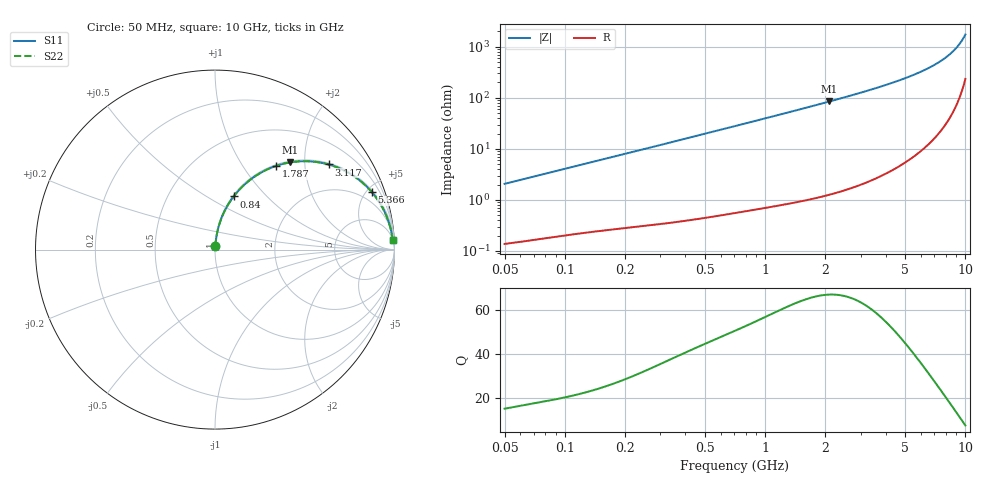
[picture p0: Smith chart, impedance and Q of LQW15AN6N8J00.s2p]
!Murata Part Number: LQW15AN6N8J00
!These Parameters are Measured in Series Mode Connection
!  o--[Z]--o
!Port1  Port2
!  o-------o
!Freq. Start=50[MHz] Stop=10[GHz], 401[Steps]
# Hz S RI R 50
!Freq.(Hz)	S 11(Real)	S 11(Imag)	S 21(Real)	S 21(Imag)	S 12(Real)	S 12(Imag)	S 22(Real)	S 22(Imag)
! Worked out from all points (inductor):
!   401 points, 50 MHz to 10 GHz, reference 50 ohm
!   read as one part in series: L = 6.54 nH near 51.34 MHz
!   highest Q = 67 at 2.095 GHz (marker M1), where L = 6.45 nH
!   S11 on the Smith chart (normalised r, x): 50 MHz: 1.00, +0.04; 840 MHz: 1.01, +0.66; 1.787 GHz: 1.02, +1.44; 3.117 GHz: 1.04, +2.64; 5.366 GHz: 1.13, +5.40; 10 GHz: 6, +35
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5e7  0.0018 0.0206  0.9982 -0.0206  0.9982 -0.0206  0.0018 0.0206
1.214486e8  0.00462 0.0487  0.9954 -0.0487  0.9954 -0.0487  0.00462 0.0487
2.949953e8  0.0168 0.115  0.9832 -0.115  0.9832 -0.115  0.0168 0.115
4.628099e8  0.0364 0.1761  0.9636 -0.1761  0.9636 -0.1761  0.0364 0.1761
7.071068e8  0.077 0.2568  0.923 -0.2568  0.923 -0.2568  0.077 0.2568
8.399791e8  0.104 0.296  0.896 -0.296  0.896 -0.296  0.104 0.296
1.21714e9  0.1933 0.3867  0.8067 -0.3867  0.8067 -0.3867  0.1933 0.3867
1.717543e9  0.3241 0.4605  0.6759 -0.4605  0.6759 -0.4605  0.3241 0.4605
1.787167e9  0.3422 0.4669  0.6578 -0.4669  0.6578 -0.4669  0.3422 0.4669
2.095058e9  0.4199 0.4861  0.5801 -0.4861  0.5801 -0.4861  0.4199 0.4861
2.555552e9  0.5254 0.4918  0.4746 -0.4918  0.4746 -0.4918  0.5254 0.4918
3.117263e9  0.6327 0.4742  0.3673 -0.4742  0.3673 -0.4742  0.6327 0.4742
4.171863e9  0.7761 0.4075  0.2239 -0.4075  0.2239 -0.4075  0.7761 0.4075
5.365732e9  0.8736 0.3205  0.1264 -0.3205  0.1264 -0.3205  0.8736 0.3205
6.632392e9  0.9326 0.2348  0.0674 -0.2348  0.0674 -0.2348  0.9326 0.2348
7.276762e9  0.9518 0.1953  0.0482 -0.1953  0.0482 -0.1953  0.9518 0.1953
7.878683e9  0.9652 0.1609  0.0348 -0.1609  0.0348 -0.1609  0.9652 0.1609
8.418147e9  0.9743 0.1319  0.0257 -0.1319  0.0257 -0.1319  0.9743 0.1319
8.876195e9  0.9802 0.1086  0.0198 -0.1086  0.0198 -0.1086  0.9802 0.1086
9.236013e9  0.9838 0.091  0.0162 -0.091  0.0162 -0.091  0.9838 0.091
9.738562e9  0.9877 0.0676  0.0123 -0.0676  0.0123 -0.0676  0.9877 0.0676
1e10  0.9892 0.0558  0.0108 -0.0558  0.0108 -0.0558  0.9892 0.0558
